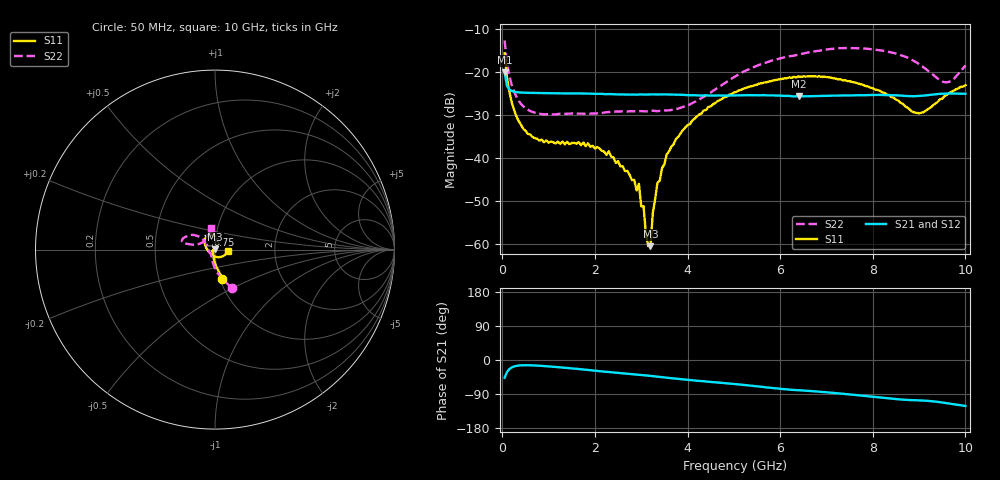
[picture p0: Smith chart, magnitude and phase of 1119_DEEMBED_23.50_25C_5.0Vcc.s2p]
!Hittite Microwave Corp.
!Digital Attenuator/PhaseShifter Rev 1.4.0
!Filename: C:\DATA\DATA\1119_DEEMBED_23.50_25C_5.0Vcc.s2p
!VNA ID: Agilent Technologies,N5224A,MY51441122,A.10.45.03
!Device type:
!2 Port Calibration.
!Temp(C): 25
!Lot Number:
!Serial Number:
!Operator:
!Misc:
!Attenuator:  23.500
# GHZ S DB R 50.0
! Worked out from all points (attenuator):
!   200 points, 50 MHz to 10 GHz, reference 50 ohm
!   highest |S21| = -19.99 dB at 50 MHz (marker M1); lowest = -25.6 dB at 6.4 GHz (marker M2)
!   lowest |S11| = -60.6 dB at 3.2 GHz (marker M3), VSWR 1.00, Z = 50 + j0.0934 ohm
!   |S11| at or under -10 dB: start of sweep to end of sweep
!   |S22| runs from -29.8 to -12.6 dB; largest |S21 - S12| = 0.00019
!   S11 on the Smith chart (normalised r, x): 50 MHz: 1.03, -0.34; 6.75 GHz: 0.91, +0.15; 10 GHz: 1.15, -0.02
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0.05  -15.57 -75.5  -19.99 -46.9  -20.00 -46.9  -12.60 -66.7
0.2  -26.86 -99.6  -24.37 -19.9  -24.37 -19.8  -22.83 -100.2
0.45  -33.18 -118.0  -24.77 -13.8  -24.77 -13.9  -27.92 -120.8
0.9  -36.34 -139.4  -24.88 -15.9  -24.88 -15.9  -29.81 -135.2
1.75  -36.37 -148.5  -24.98 -25.1  -24.98 -25.1  -29.68 -139.9
2.3  -38.44 -150.4  -25.10 -31.7  -25.09 -31.7  -29.29 -148.2
2.9  -47.59 -115.7  -25.24 -38.3  -25.25 -38.4  -29.06 -157.8
2.95  -46.02 -124.9  -25.20 -38.9  -25.20 -38.9  -29.09 -158.9
3.15  -60.54 -89.7  -25.20 -41.2  -25.21 -41.2  -29.09 -164.8
3.2  -60.56 84.6  -25.18 -41.9  -25.19 -41.9  -29.09 -166.2
3.25  -52.84 54.2  -25.17 -42.6  -25.18 -42.7  -28.98 -167.6
3.4  -45.29 71.8  -25.19 -44.5  -25.20 -44.5  -29.02 -172.3
3.55  -39.17 69.2  -25.19 -46.8  -25.20 -46.8  -28.92 -177.7
3.9  -33.50 66.6  -25.28 -51.2  -25.29 -51.2  -28.11 168.0
5.05  -24.62 81.3  -25.41 -63.7  -25.42 -63.8  -20.86 139.4
6.4  -20.96 107.9  -25.65 -79.7  -25.67 -79.7  -15.90 150.5
6.7  -20.98 114.7  -25.57 -82.3  -25.58 -82.3  -15.21 154.5
6.75  -20.92 115.1  -25.57 -82.9  -25.58 -82.9  -15.12 155.1
8.35  -25.33 163.4  -25.35 -101.2  -25.36 -101.2  -15.26 168.2
8.999999  -29.57 -130.0  -25.54 -106.5  -25.55 -106.5  -18.13 167.4
9.6  -25.27 -46.3  -25.00 -114.1  -25.01 -114.1  -22.35 133.4
10  -23.02 -7.7  -25.03 -121.4  -25.03 -121.3  -18.42 99.7
